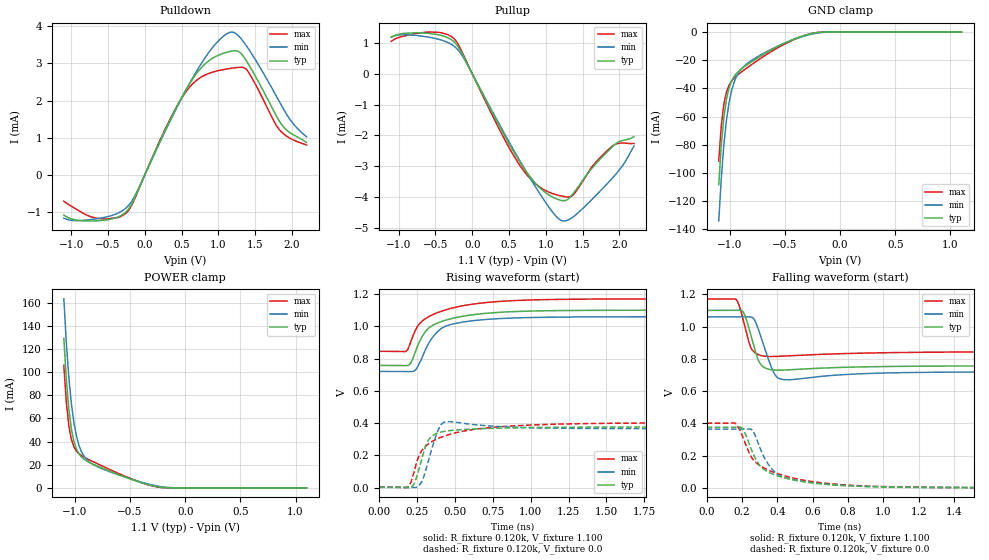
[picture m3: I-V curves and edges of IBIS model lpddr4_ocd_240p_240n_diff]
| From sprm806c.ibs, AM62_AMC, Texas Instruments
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|   Model lpddr4_ocd_240p_240n_diff
[Model] lpddr4_ocd_240p_240n_diff
Model_type I/O
Polarity   Non-Inverting
Enable   Active-High
Vinl =  0.113V
Vinh =  0.253V
Vmeas =  0.183V
C_comp   2.935pF   2.458pF   2.940pF
[Model Spec]
Vinh   0.253V   0.247V   0.265V
Vinl   0.113V   0.107V   0.125V
Vmeas   0.183V   0.176V   0.195V
[Temperature Range]   25.000   0.125k   -40.000
[Voltage Range]   1.100V   1.060V   1.170V
[Pullup Reference]   1.100V   1.060V   1.170V
[Pulldown Reference]   0.0V   0.0V   0.0V
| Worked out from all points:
|   slope of the pulldown table from 0 to 0.165 V, typ, clamps not added: 226 ohm
|   slope of the pullup table from 0 to 0.165 V, typ, clamps not added: 214 ohm
|   GND clamp passes 1 mA (typ) near -0.25 V on its own axis
|   POWER clamp passes 1 mA (typ) near -0.26 V on its own axis
|   rising waveform, R_fixture 0.120k, V_fixture 1.100: 20-80 % time 185ps typ, 144ps min, 239ps max; typ from 0.757 V to 1.1 V
|   rising waveform, R_fixture 0.120k, V_fixture 0.0: 20-80 % time 79.3ps typ, 67.3ps min, 212ps max; typ from 0.001 V to 0.376 V
|   falling waveform, R_fixture 0.120k, V_fixture 1.100: 20-80 % time 54.1ps typ, 62.7ps min, 46.1ps max; typ from 1.1 V to 0.757 V
|   falling waveform, R_fixture 0.120k, V_fixture 0.0: 20-80 % time 168ps typ, 132ps min, 218ps max; typ from 0.376 V to 0.001 V
[Pulldown]
|Voltage   I(typ)   I(min)   I(max)
-1.1V     -1.073mA   -1.157mA   -700.5uA
-658mV    -1.228mA   -1.173mA   -1.155mA
-249mV    -978.8uA   -873.8uA   -1.012mA
-113mV    -509.6uA   -474.3uA   -526.3uA
329mV     1.421mA    1.384mA    1.44mA
567mV     2.313mA    2.306mA    2.256mA
839mV     3.017mA    3.205mA    2.702mA
1.145V    3.313mA    3.823mA    2.858mA
1.281V    3.312mA    3.725mA    2.892mA
1.384V    3.063mA    3.466mA    2.835mA
1.826V    1.461mA    1.987mA    1.228mA
2.2V      874uA      1.029mA    805.9uA
[Pullup]
|Voltage   I(typ)   I(min)   I(max)
-1.1V     1.175mA    1.195mA    1.049mA
-590mV    1.307mA    1.183mA    1.35mA
-249mV    1.038mA    895.4uA    1.14mA
-113mV    537.4uA    496.1uA    574.8uA
397mV     -1.824mA   -1.763mA   -1.933mA
669mV     -2.942mA   -2.912mA   -3.047mA
941mV     -3.747mA   -3.971mA   -3.713mA
1.213V    -4.113mA   -4.761mA   -3.966mA
1.384V    -3.852mA   -4.625mA   -3.905mA
1.622V    -3.083mA   -4.091mA   -3.033mA
1.894V    -2.395mA   -3.417mA   -2.372mA
2.2V      -2.041mA   -2.34mA    -2.262mA
[GND_clamp]
|Voltage   I(typ)   I(min)   I(max)
-1.1V     -108.4mA   -134.2mA   -91.64mA
-1.077V   -80.17mA   -103.9mA   -66.63mA
-1.054V   -60.68mA   -80.47mA   -51.43mA
-1.031V   -48.01mA   -63.16mA   -42.83mA
-1.008V   -40.05mA   -50.75mA   -37.96mA
-985mV    -35.04mA   -42.04mA   -34.98mA
-940mV    -29.42mA   -31.64mA   -31.22mA
-894mV    -26.11mA   -26.16mA   -28.35mA
-848mV    -23.5mA    -22.73mA   -25.7mA
-527mV    -8.739mA   -8.686mA   -9.514mA
-229mV    -630.6uA   -1.042mA   -565.5uA
1.1V      0A         0A         0A
[POWER_clamp]
|Voltage   I(typ)   I(min)   I(max)
-1.1V     129.2mA    163.4mA    105.9mA
-1.077V   92.86mA    124.8mA    73.4mA
-1.054V   67.3mA     94.73mA    53.17mA
-1.031V   50.48mA    72.25mA    41.67mA
-1.008V   39.92mA    56.03mA    35.37mA
-985mV    33.38mA    44.6mA     31.76mA
-963mV    29.31mA    36.69mA    29.53mA
-917mV    24.75mA    27.38mA    26.61mA
-871mV    22.09mA    22.57mA    24.31mA
-619mV    11.98mA    11.76mA    13.12mA
-229mV    602.7uA    1.183mA    400.7uA
1.1V      0A         0A         0A
[Ramp]
| variable   typ   min   max
dV/dt_r   0.225/78.731p   0.217/67.340p   0.240/0.213n
dV/dt_f   0.206/53.581p   0.204/62.155p   0.195/45.916p
R_load = 0.120k
[Rising Waveform]
R_fixture= 0.120k
V_fixture= 1.100
V_fixture_min= 1.060
V_fixture_max= 1.170
|time   V(typ)   V(min)   V(max)
0s        757.2mV    720mV      844.7mV
177ps     756.1mV    719.9mV    844.2mV
209ps     772.1mV    719.2mV    906.4mV
232ps     825.1mV    722.6mV    959.9mV
267ps     907.3mV    772.6mV    1.017V
314ps     977.8mV    871.6mV    1.053V
395ps     1.024V     975.1mV    1.088V
615ps     1.071V     1.034V     1.137V
1.18ns    1.097V     1.057V     1.167V
3ns       1.1V       1.059V     1.17V
[Rising Waveform]
R_fixture= 0.120k
V_fixture= 0.0
V_fixture_min= 0.0
V_fixture_max= 0.0
|time   V(typ)   V(min)   V(max)
0s        1.441mV    2.65mV     2.438mV
192ps     -1.237mV   1.741mV    4.817mV
230ps     22.63mV    392.5uV    94.48mV
261ps     108.5mV    11.17mV    193.8mV
293ps     216.3mV    62.89mV    243.2mV
322ps     290.8mV    156.1mV    269.1mV
395ps     340.7mV    368mV      307mV
442ps     350.2mV    407.7mV    323.2mV
1.1ns     373mV      369.3mV    391.1mV
3ns       376mV      364.9mV    402mV
[Falling Waveform]
R_fixture= 0.120k
V_fixture= 1.100
V_fixture_min= 1.060
V_fixture_max= 1.170
|time   V(typ)   V(min)   V(max)
0s        1.1V       1.059V     1.17V
169ps     1.101V     1.059V     1.165V
208ps     1.088V     1.06V      1.036V
261ps     904.7mV    1.055V     850.3mV
293ps     789mV      982.5mV    825.6mV
313ps     756.9mV    915.1mV    819.1mV
385ps     730.3mV    702.7mV    814.6mV
441ps     730.4mV    670.6mV    817.1mV
1.11ns    753.6mV    714.5mV    839.3mV
3ns       757.2mV    719.8mV    844.7mV
[Falling Waveform]
R_fixture= 0.120k
V_fixture= 0.0
V_fixture_min= 0.0
V_fixture_max= 0.0
|time   V(typ)   V(min)   V(max)
0s        375.9mV    364.9mV    401.8mV
162ps     376.5mV    364.9mV    401.2mV
206ps     362.8mV    365.7mV    311.5mV
251ps     243.7mV    364.9mV    195.5mV
308ps     129.8mV    231.6mV    134.6mV
358ps     93.75mV    132.7mV    107.1mV
401ps     75.85mV    85.35mV    89.32mV
645ps     26.37mV    26.74mV    33.31mV
1.184ns   3.964mV    5.049mV    5.533mV
3ns       1.431mV    2.627mV    2.433mV
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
